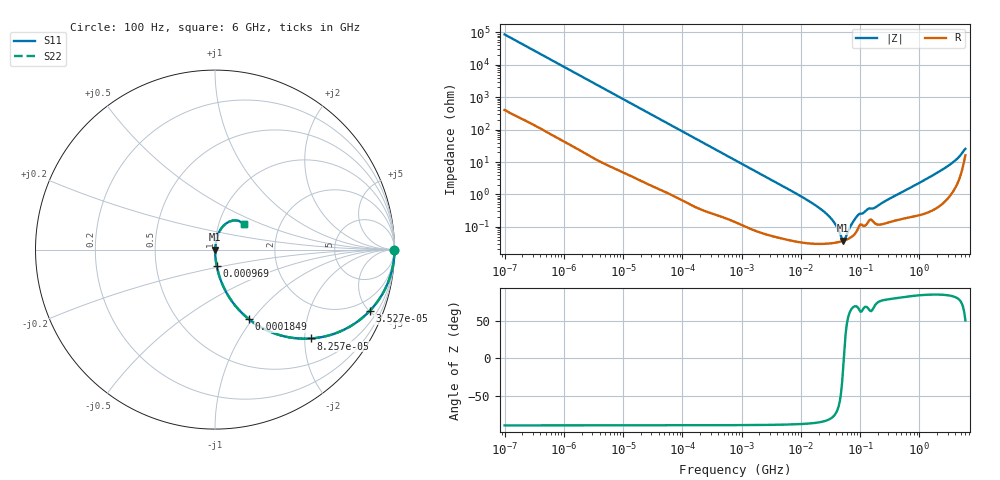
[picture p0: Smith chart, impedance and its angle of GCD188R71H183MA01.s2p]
!Murata Part Number: GCD188R71H183MA01
!These Parameters are Measured in Series Mode Connection
!Data Generated on Mar 13, 2026
!  o--ll--o
!Port1  Port2
!  o------o
!Operation Temp=25[degC], DC Bias Voltage=0[V]
!Freq. Start=100[Hz] Stop=6[GHz] 401[Steps]
# Hz S RI R 50
!Freq.(Hz) S11(Real) S11(Imag) S21(Real) S21(Imag) S12(Real) S12(Imag) S22(Real) S22(Imag)
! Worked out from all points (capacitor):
!   401 points, 100 Hz to 6 GHz, reference 50 ohm
!   read as one part in series: C = 18.3 nF near 109 Hz
!   lowest |Z| = 37.5 mohm at 52.11 MHz (marker M1)
!   series resonance near 53.13 MHz, so ESL is about 490 pH
!   S11 on the Smith chart (normalised r, x): 100 Hz: open; 35.27 kHz: 1.03, -5.01; 82.57 kHz: 1.02, -2.15; 184.9 kHz: 1.01, -0.96; 969 kHz: 1.00, -0.19; 6 GHz: 1.32, +0.39
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100  1 -0.00115  6.7e-06 0.00115  6.7e-06 0.00115  1 -0.00115
2008  0.9994 -0.0229  0.000638 0.0229  0.000638 0.0229  0.9994 -0.0229
10066  0.9865 -0.1128  0.0135 0.1128  0.0135 0.1128  0.9865 -0.1128
35265  0.861 -0.3427  0.139 0.3427  0.139 0.3427  0.861 -0.3427
40335  0.8261 -0.3757  0.1739 0.3757  0.1739 0.3757  0.8261 -0.3757
82567  0.5356 -0.4951  0.4644 0.4951  0.4644 0.4951  0.5356 -0.4951
184852  0.1901 -0.3885  0.8099 0.3885  0.8099 0.3885  0.1901 -0.3885
330837  0.0698 -0.2502  0.9302 0.2502  0.9302 0.2502  0.0698 -0.2502
774597  0.0146 -0.114  0.9854 0.114  0.9854 0.114  0.0146 -0.114
968953  0.00967 -0.0917  0.9903 0.0917  0.9903 0.0917  0.00967 -0.0917
1.555665e7  0.00033 -0.00537  0.9997 0.00537  0.9997 0.00537  0.00033 -0.00537
3.184506e7  0.000311 -0.00185  0.9997 0.00185  0.9997 0.00185  0.000311 -0.00185
3.80911e7  0.000323 -0.00117  0.9997 0.00117  0.9997 0.00117  0.000323 -0.00117
4.764863e7  0.000352 -0.000379  0.9996 0.000379  0.9996 0.000379  0.000352 -0.000379
5.211241e7  0.000369 -6.7e-05  0.9996 6.7e-05  0.9996 6.7e-05  0.000369 -6.7e-05
5.699437e7  0.000391 0.000247  0.9996 -0.000247  0.9996 -0.000247  0.000391 0.000247
7.455971e7  0.000514 0.00124  0.9995 -0.00124  0.9995 -0.00124  0.000514 0.00124
9.326766e7  0.00091 0.00216  0.9991 -0.00216  0.9991 -0.00216  0.00091 0.00216
3.124326e8  0.00144 0.00719  0.9986 -0.00719  0.9986 -0.00719  0.00144 0.00719
2.450438e9  0.00837 0.0572  0.9916 -0.0572  0.9916 -0.0572  0.00837 0.0572
4.385646e9  0.0355 0.1189  0.9645 -0.1189  0.9645 -0.1189  0.0355 0.1189
6e9  0.1631 0.1422  0.8369 -0.1422  0.8369 -0.1422  0.1631 0.1422
